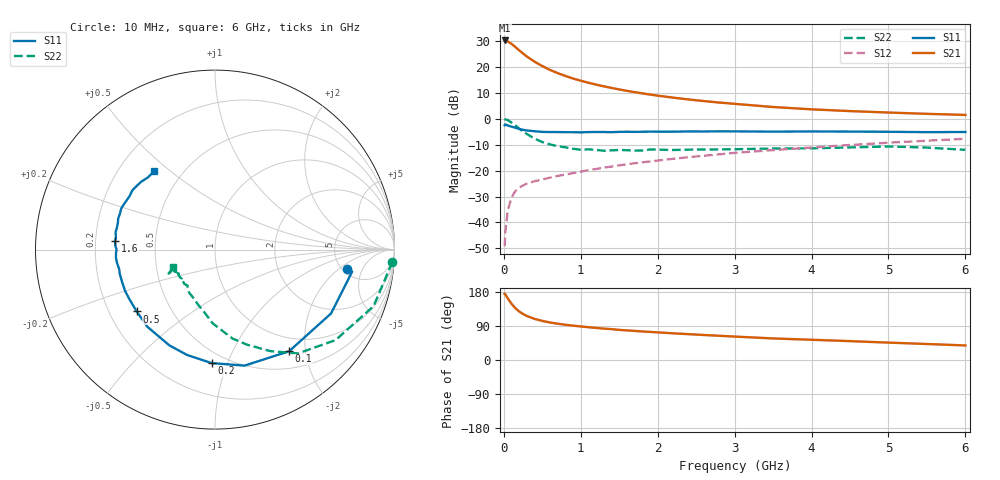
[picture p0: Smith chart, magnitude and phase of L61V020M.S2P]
!  INFINEON TECHNOLOGIES Small Signal Semiconductors
! BFR380L3 , Si-NPN RF-Transistor in TSLP-3-1
!  Vce=1 V,  Ic=20 mA
! Common Emitter S-Parameters:  07. March 2005
#  GHz  S  MA  R  50
! f  S11  S21  S12  S22
! GHz  Mag  Ang  Mag  Ang  Mag  Ang  Mag  Ang
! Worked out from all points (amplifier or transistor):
!   36 points, 10 MHz to 6 GHz, reference 50 ohm
!   highest |S21| = 30.1 dB at 10 MHz (marker M1)
!   |S21| within 3 dB of that: start of sweep to 168 MHz
!   unconditionally stable (mu >= 1): 1.819 GHz to 5.036 GHz
!   at 250 MHz: K = 0.37, MSG = 25.4 dB, |S12| = -25.7 dB
!   at 1.4 GHz: K = 0.96, MSG = 15.1 dB, |S12| = -18.5 dB
!   at 6 GHz: K = 0.99, MSG = 4.6 dB, |S12| = -7.8 dB
!   S11 on the Smith chart (normalised r, x): 10 MHz: 5.52, -2.67; 100 MHz: 0.76, -1.70; 200 MHz: 0.42, -0.88; 500 MHz: 0.32, -0.32; 1.6 GHz: 0.28, +0.04; 6 GHz: 0.35, +0.44
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0.01  0.745 -8.3  32.01 174.7  0.0035 82.9  0.9898 -4.0
0.02  0.774 -9.1  31.9 173.2  0.0066 85.4  0.9694 -8.1
0.05  0.7381 -28.8  30.7 162.9  0.0167 78.4  0.9382 -19.6
0.1  0.7009 -53.9  27.5 148.4  0.0305 66.4  0.8399 -36.9
0.15  0.6671 -75.7  23.91 136.6  0.0404 58.3  0.7404 -51.4
0.2  0.6325 -91.7  20.62 127.9  0.0467 54.8  0.6443 -61.4
0.25  0.6076 -104.7  17.94 121.4  0.0518 51.0  0.559 -71.4
0.3  0.5912 -115.4  15.66 116.1  0.0562 49.5  0.5055 -78.8
0.4  0.5717 -131.2  12.47 108.4  0.0625 47.8  0.4117 -91.7
0.5  0.5559 -141.7  10.28 103.2  0.0671 48.3  0.3537 -99.7
0.6  0.5512 -149.8  8.657 99.0  0.0732 49.2  0.3198 -107.4
0.8  0.5479 -161.2  6.636 93.0  0.0838 52.1  0.2801 -120.8
0.9  0.5475 -165.9  5.914 90.6  0.0892 53.5  0.2627 -125.7
1.1  0.5505 -172.0  4.907 86.5  0.1018 55.6  0.2565 -131.7
1.3  0.5521 -178.0  4.192 82.8  0.1139 57.0  0.2409 -139.4
1.6  0.5597 175.0  3.428 78.1  0.1321 58.6  0.2467 -146.0
2.2  0.5605 165.1  2.538 70.4  0.1686 60.4  0.2488 -149.2
2.8  0.5702 156.4  2.041 63.9  0.2052 61.1  0.2555 -154.4
3.5  0.5615 147.8  1.674 56.9  0.2474 59.7  0.2657 -153.7
4.5  0.5628 141.3  1.397 49.8  0.311 58.5  0.2791 -153.3
5.5  0.549 132.8  1.237 42.2  0.3758 54.8  0.2767 -154.0
6  0.5529 127.8  1.179 38.4  0.4089 52.7  0.2507 -157.8
